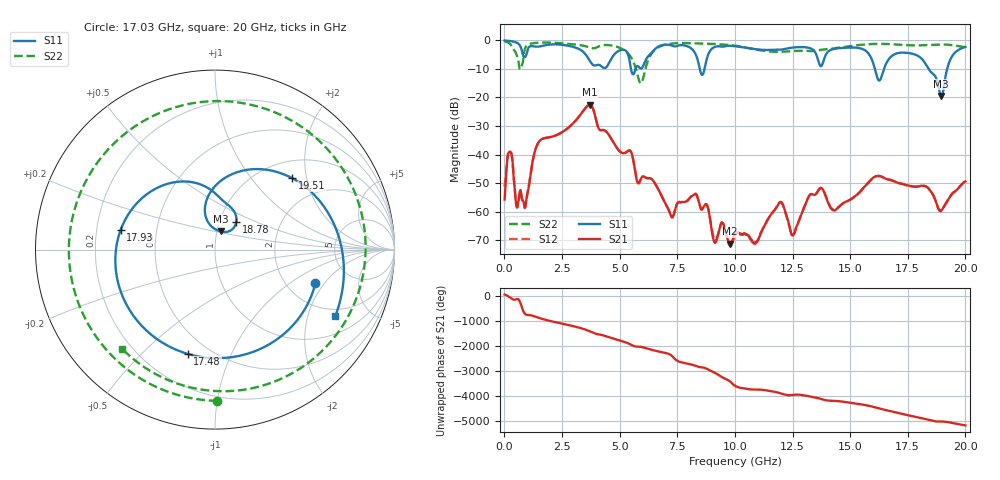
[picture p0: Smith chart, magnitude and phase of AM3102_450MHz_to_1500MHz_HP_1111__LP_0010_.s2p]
!Agilent Technologies,E8364B,MY43040894,A.07.50.67
!Agilent E8364B: A.07.50.67
!Date: Thursday, January 11, 2018 06:49:05
!Correction: S11(Full 2 Port(1,2))
!S21(Full 2 Port(1,2))
!S12(Full 2 Port(1,2))
!S22(Full 2 Port(1,2))
!S2P File: Measurements: S11, S21, S12, S22:
# Hz S  dB  R 50
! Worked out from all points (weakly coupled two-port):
!   1601 points, 10 MHz to 20 GHz, reference 50 ohm
!   highest |S21| = -22.58 dB at 3.708 GHz (marker M1); lowest = -71.2 dB at 9.793 GHz (marker M2)
!   lowest |S11| = -19.5 dB at 18.95 GHz (marker M3), VSWR 1.24, Z = 52.1 + j10.6 ohm
!   |S11| at or under -10 dB: 8.477 GHz to 8.684 GHz (206.6 MHz wide, 2.41 % of centre); 16.07 GHz to 16.47 GHz (396.6 MHz wide, 2.44 % of centre); 18.4 GHz to 19.21 GHz (808.4 MHz wide, 4.3 % of centre)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
!   |S22| runs from -15.1 to -0.3 dB; largest |S21 - S12| = 0.0013
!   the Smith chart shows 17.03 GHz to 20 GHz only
!   S11 on the Smith chart (normalised r, x): 17.03 GHz: 2.83, -1.64; 17.48 GHz: 0.38, -0.70; 17.93 GHz: 0.30, +0.09; 18.78 GHz: 1.20, +0.38; 19.51 GHz: 1.36, +1.65; 20 GHz: 1.68, -3.01
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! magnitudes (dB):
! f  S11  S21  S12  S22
! 10 MHz  -0.1  -55.7  -51.2  -0.3
! 247.4 MHz  -0.3  -39.0  -39.0  -1.3
! 872.1 MHz  -5.9  -58.4  -58.4  -3.6
! 1.484 GHz  -2.2  -35.7  -35.7  -0.9
! 3.346 GHz  -3.6  -25.5  -25.5  -1.8
! 3.708 GHz  -7.2  -22.6  -22.6  -2.6
! 5.92 GHz  -9.9  -48.6  -48.6  -15.1
! 6.682 GHz  -2.2  -52.2  -52.2  -2.4
! 8.581 GHz  -12.1  -59.1  -59.2  -1.2
! 9.793 GHz  -1.9  -71.2  -71.9  -1.7
! 10.01 GHz  -2.1  -67.6  -67.9  -1.9
! 11.98 GHz  -3.3  -56.6  -56.7  -4.0
! 12.53 GHz  -2.5  -68.3  -67.9  -3.8
! 13.34 GHz  -3.1  -53.8  -53.8  -3.8
! 16.68 GHz  -6.6  -48.7  -48.8  -1.3
! 17.03 GHz  -4.6  -49.7  -49.8  -1.5
! 17.48 GHz  -4.4  -50.7  -50.8  -1.7
! 17.93 GHz  -5.4  -51.2  -51.1  -1.8
! 18.78 GHz  -14.3  -57.8  -57.8  -1.5
! 18.95 GHz  -19.5  -59.5  -59.7  -1.5
! 19.51 GHz  -4.6  -53.1  -53.1  -1.8
! 20 GHz  -2.3  -49.4  -49.4  -2.4
